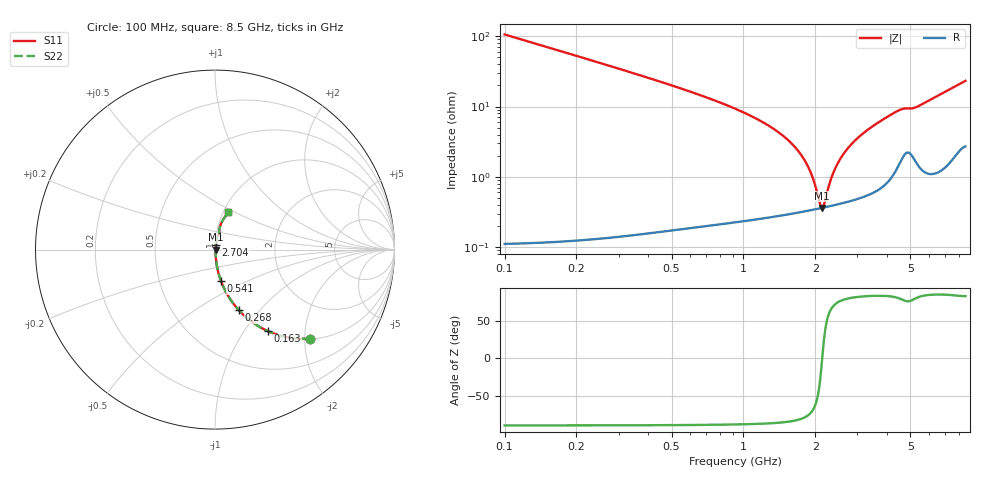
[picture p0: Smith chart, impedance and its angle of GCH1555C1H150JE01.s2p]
!Murata Part Number: GCH1555C1H150JE01
!These Parameters are Measured in Series Mode Connection
!Data Generated on Mar 13, 2026
!  o--ll--o
!Port1  Port2
!  o------o
!Operation Temp=25[degC], DC Bias Voltage=0[V]
!Freq. Start=100[MHz] Stop=9[GHz] 401[Steps]
# Hz S RI R 50
!Freq.(Hz) S11(Real) S11(Imag) S21(Real) S21(Imag) S12(Real) S12(Imag) S22(Real) S22(Imag)
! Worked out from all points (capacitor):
!   401 points, 100 MHz to 8.5 GHz, reference 50 ohm
!   read as one part in series: C = 15 pF near 142 MHz
!   lowest |Z| = 362 mohm at 2.137 GHz (marker M1)
!   series resonance near 2.137 GHz, so ESL is about 370 pH
!   S11 on the Smith chart (normalised r, x): 100 MHz: 1.00, -2.12; 163 MHz: 1.00, -1.29; 268 MHz: 1.00, -0.78; 541 MHz: 1.00, -0.37; 2.704 GHz: 1.01, +0.05; 8.5 GHz: 1.05, +0.46
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1e8  0.5284 -0.4987  0.4716 0.4987  0.4716 0.4987  0.5284 -0.4987
1.63e8  0.2953 -0.4553  0.7047 0.4553  0.7047 0.4553  0.2953 -0.4553
2.68e8  0.1324 -0.3373  0.8676 0.3373  0.8676 0.3373  0.1324 -0.3373
5.41e8  0.0341 -0.1766  0.9659 0.1766  0.9659 0.1766  0.0341 -0.1766
9.19e8  0.0109 -0.0926  0.9891 0.0926  0.9891 0.0926  0.0109 -0.0926
1.507e9  0.00412 -0.0351  0.9959 0.0351  0.9959 0.0351  0.00412 -0.0351
1.696e9  0.00362 -0.023  0.9964 0.023  0.9964 0.023  0.00362 -0.023
1.843e9  0.00348 -0.0147  0.9965 0.0147  0.9965 0.0147  0.00348 -0.0147
1.948e9  0.00347 -0.00917  0.9965 0.00917  0.9965 0.00917  0.00347 -0.00917
2.095e9  0.00356 -0.00197  0.9964 0.00197  0.9964 0.00197  0.00356 -0.00197
2.137e9  0.00361 -1.2e-05  0.9964 1.2e-05  0.9964 1.2e-05  0.00361 -1.2e-05
2.179e9  0.00366 0.00191  0.9963 -0.00191  0.9963 -0.00191  0.00366 0.00191
2.305e9  0.00387 0.00749  0.9961 -0.00749  0.9961 -0.00749  0.00387 0.00749
2.41e9  0.00409 0.0119  0.9959 -0.0119  0.9959 -0.0119  0.00409 0.0119
2.536e9  0.00441 0.0171  0.9956 -0.0171  0.9956 -0.0171  0.00441 0.0171
2.704e9  0.00491 0.0236  0.9951 -0.0236  0.9951 -0.0236  0.00491 0.0236
2.914e9  0.00567 0.0315  0.9943 -0.0315  0.9943 -0.0315  0.00567 0.0315
3.481e9  0.00853 0.0515  0.9915 -0.0515  0.9915 -0.0515  0.00853 0.0515
4.3e9  0.0177 0.0792  0.9823 -0.0792  0.9823 -0.0792  0.0177 0.0792
5.707e9  0.0234 0.1073  0.9766 -0.1073  0.9766 -0.1073  0.0234 0.1073
7.114e9  0.0401 0.1577  0.9599 -0.1577  0.9599 -0.1577  0.0401 0.1577
8.5e9  0.0729 0.2077  0.9271 -0.2077  0.9271 -0.2077  0.0729 0.2077
